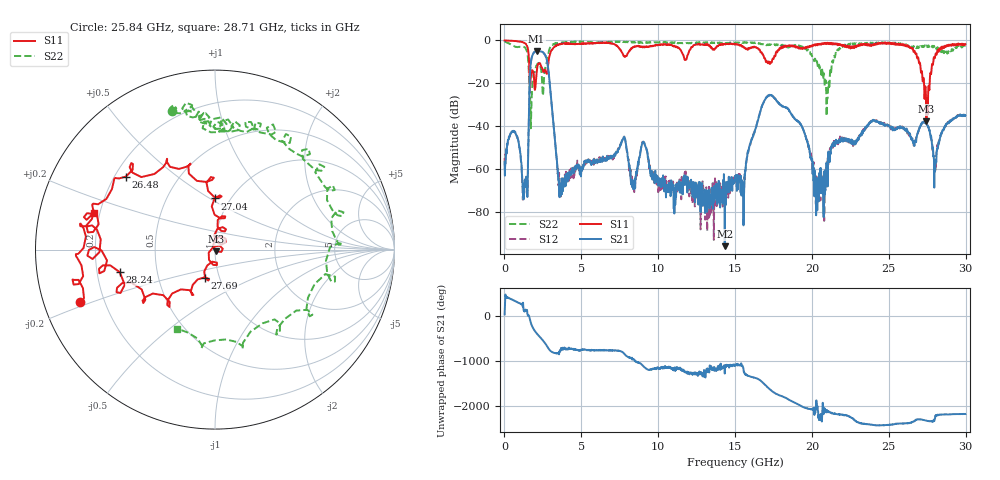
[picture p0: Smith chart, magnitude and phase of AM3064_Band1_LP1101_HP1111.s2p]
# Hz S DB R 50.0
!freq dBS11 angS11 dBS21 angS21 dBS12 angS12 dBS22 angS22
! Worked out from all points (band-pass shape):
!   1600 points, 10 MHz to 29.98 GHz, reference 50 ohm
!   highest |S21| = -5.00 dB at 2.091 GHz (marker M1); lowest = -96.0 dB at 14.33 GHz (marker M2)
!   |S21| within 3 dB of the highest: 1.775 GHz to 2.711 GHz (936.1 MHz wide, 41.7 % of centre)
!   lowest |S11| = -37.7 dB at 27.45 GHz (marker M3), VSWR 1.03, Z = 50.8 - j1.07 ohm
!   |S11| at or under -10 dB: 1.6 GHz to 2.859 GHz (1.259 GHz wide, 56.5 % of centre); 17.22 GHz to 17.39 GHz (173.9 MHz wide, 1 % of centre); 26.95 GHz to 27.89 GHz (940.1 MHz wide, 3.43 % of centre)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
!   |S22| runs from -41.0 to -0.4 dB; largest |S21 - S12| = 0.0088
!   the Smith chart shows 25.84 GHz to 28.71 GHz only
!   S11 on the Smith chart (normalised r, x): 25.84 GHz: 0.11, -0.19; 26.48 GHz: 0.24, +0.34; 27.04 GHz: 0.85, +0.52; 27.69 GHz: 0.85, -0.28; 28.24 GHz: 0.30, -0.11; 28.71 GHz: 0.18, +0.14
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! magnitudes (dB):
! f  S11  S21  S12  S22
! 10 MHz  0.0  -56.9  -54.9  -0.4
! 684.8 MHz  -0.3  -42.9  -43.1  -2.9
! 1.36 GHz  -1.5  -65.2  -67.2  -3.5
! 1.753 GHz  -15.1  -8.7  -8.7  -30.8
! 2.091 GHz  -15.3  -5.0  -4.9  -11.6
! 2.784 GHz  -14.8  -10.0  -10.0  -9.2
! 3.646 GHz  -1.8  -68.8  -69.7  -1.0
! 5.015 GHz  -1.4  -60.6  -60.8  -0.6
! 10 GHz  -2.1  -65.0  -70.8  -1.0
! 14.33 GHz  -1.7  -96.0  -68.7  -1.1
! 15 GHz  -1.7  -65.8  -63.2  -1.3
! 17.25 GHz  -11.0  -25.5  -25.4  -2.0
! 19.99 GHz  -2.9  -56.3  -56.7  -6.9
! 25 GHz  -1.1  -39.6  -39.6  -1.2
! 25.84 GHz  -1.9  -40.4  -40.8  -1.8
! 26.48 GHz  -3.9  -46.2  -46.3  -2.9
! 27.04 GHz  -10.9  -40.3  -40.2  -3.4
! 27.45 GHz  -37.7  -38.9  -38.8  -2.4
! 27.69 GHz  -15.5  -43.8  -44.0  -2.3
! 28.24 GHz  -5.3  -47.4  -48.6  -4.7
! 28.71 GHz  -3.0  -39.2  -39.9  -6.2
! 29.98 GHz  -1.8  -34.9  -35.2  -2.9
